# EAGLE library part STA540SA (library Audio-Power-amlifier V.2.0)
4 x 10W DUAL/QUAD POWER AMPLIFIER
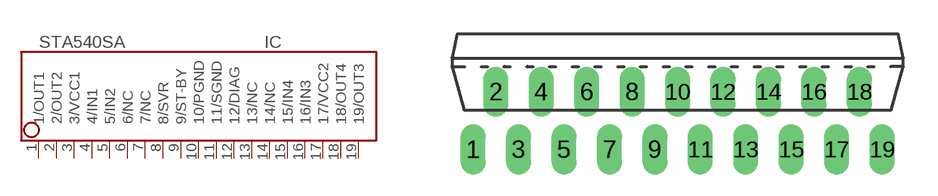
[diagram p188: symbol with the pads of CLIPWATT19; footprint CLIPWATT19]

Designator prefix IC

## STA540SA  [CLIPWATT19]
1  1/OUT1  out
2  2/OUT2  out
3  3/VCC1  pwr
4  4/IN1  in
5  5/IN2  in
6  6/NC  nc
7  7/NC  nc
8  8/SVR  in
9  9/ST-BY  in
10  10/PGND  pwr
11  11/SGND  pwr
12  12/DIAG  out
13  13/NC  nc
14  14/NC  nc
15  15/IN4  in
16  16/IN3  in
17  17/VCC2  pwr
18  18/OUT4  out
19  19/OUT3  out

## Footprint CLIPWATT19 (pad centres in mm)
CLIPWATT 19
drill 0.6 long: 1 -9,-2.54; 2 -8,0; 3 -7,-2.54; 4 -6,0; 5 -5,-2.54; 6 -4,0; 7 -3,-2.54; 8 -2,0; 9 -1,-2.54; 10 0,0; 11 1,-2.54; 12 2,0; 13 3,-2.54; 14 4,0; 15 5,-2.54; 16 6,0; 17 7,-2.54; 18 8,0; 19 9,-2.54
